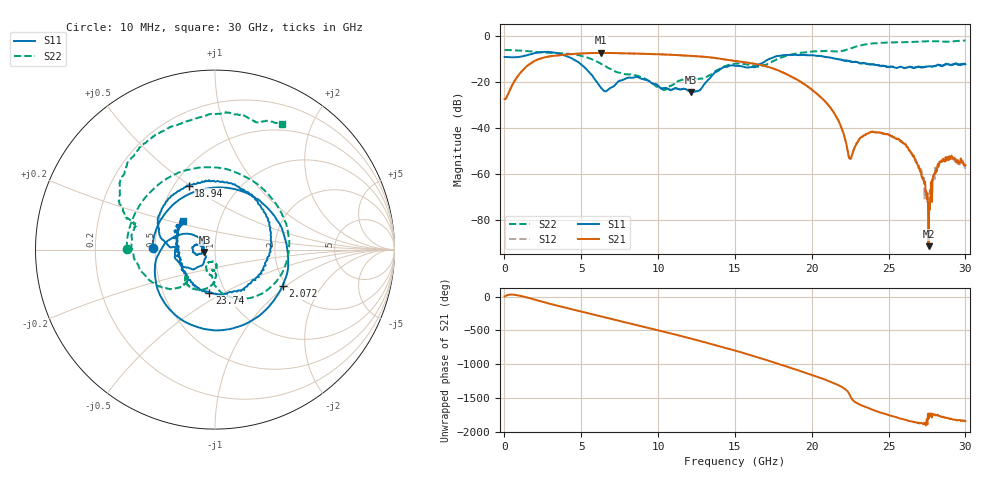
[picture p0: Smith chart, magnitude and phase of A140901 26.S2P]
!  2-Port S-parameters saved by WinCal
! VAR MeasName=S-Parameters (CALIBRATED_DATA) read from VNA (N5244A)
! VAR MeasDate=11/3/2014 9:28:58 AM
! VAR NAME=A140901 26
! VAR FILENAME=A140901 26.S2P
! VAR DATE=11/3/2014 9:28:58 AM
! VAR PHYS_PORTS=1,2
# Hz S RI R 50
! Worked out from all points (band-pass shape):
!   801 points, 10 MHz to 30 GHz, reference 50 ohm
!   highest |S21| = -7.37 dB at 6.27 GHz (marker M1); lowest = -91.5 dB at 27.6 GHz (marker M2)
!   |S21| within 3 dB of the highest: 2.126 GHz to 14.45 GHz (12.32 GHz wide, 149 % of centre)
!   lowest |S11| = -24.4 dB at 12.16 GHz (marker M3), VSWR 1.13, Z = 44.4 - j1.17 ohm
!   |S11| at or under -10 dB: 4.442 GHz to 17.25 GHz (12.8 GHz wide, 118 % of centre); 21.56519 GHz to 21.61698 GHz (51.79 MHz wide, 0.24 % of centre); 21.65 GHz to end of sweep
!   |S22| runs from -23.6 to -2.0 dB; largest |S21 - S12| = 0.0026
!   S11 on the Smith chart (normalised r, x): 10 MHz: 0.48, +0.01; 2.072 GHz: 1.90, -0.94; 18.94 GHz: 0.59, +0.49; 23.74 GHz: 0.84, -0.43; 30 GHz: 0.66, +0.23
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1e7  -0.3472 0.00636  0.0421 0.00181  0.0414 0.000932  -0.4921 0.00332
1.022162e9  0.0859 0.3414  0.1517 0.0292  0.1517 0.0293  -0.2934 0.3792
2.071812e9  0.3761 -0.2015  0.186 -0.2324  0.1864 -0.2321  0.0915 0.4405
3.6088e9  -0.292 -0.2787  -0.3096 -0.221  -0.3094 -0.2213  0.4008 0.1256
5.033325e9  -0.2213 0.0739  -0.3004 0.2876  -0.2995 0.2877  0.2864 -0.2292
6.270412e9  -0.0681 0.0321  0.1628 0.396  0.1626 0.3955  0.0423 -0.2455
7.8074e9  -0.1129 -0.0219  0.3996 -0.1201  0.399 -0.1196  -0.0158 -0.1473
1.001916e10  -0.079 0.0206  -0.3016 -0.2615  -0.3011 -0.2609  -0.0318 -0.0689
1.215595e10  -0.0586 -0.0131  -0.0477 0.3645  -0.0482 0.3637  -0.0122 -0.1171
1.358048e10  -0.1056 -0.1028  0.3294 0.0596  0.3295 0.0592  0.00401 -0.1557
1.5005e10  -0.2232 -0.023  0.0542 -0.28  0.0524 -0.2791  -0.1151 -0.2201
1.646701e10  -0.2272 0.014  -0.2401 -0.0152  -0.2402 -0.0151  -0.1522 -0.1493
1.894119e10  -0.1468 0.3559  0.1168 0.00439  0.1158 0.00473  -0.3789 -0.1562
2.002832e10  0.0912 0.3702  0.0109 -0.0657  0.0117 -0.0656  -0.4538 -0.0291
2.156531e10  0.3104 0.0605  -0.0152 0.00989  -0.0154 0.00979  -0.4388 0.1325
2.25025e10  0.2234 -0.1632  0.00193 -0.00111  0.00184 -0.00106  -0.4993 0.1801
2.373959e10  -0.0312 -0.2417  -0.00659 0.00432  -0.00662 0.00432  -0.4969 0.4426
2.501416e10  -0.1674 -0.1234  0.00491 0.00506  0.00499 0.005  -0.3328 0.6393
2.655115e10  -0.2063 -0.0279  0.00166 -0.0019  0.00178 -0.00197  -0.1043 0.7322
2.76008e10  -0.2156 0.0309  2.63e-05 -3.88e-06  -0.000168 1.88e-05  0.0628 0.7663
2.842552e10  -0.2132 0.0671  0.00168 0.000865  0.00174 0.000892  0.1989 0.7254
3e10  -0.1796 0.1602  0.00116 -0.00099  0.00115 -0.00111  0.3735 0.701
